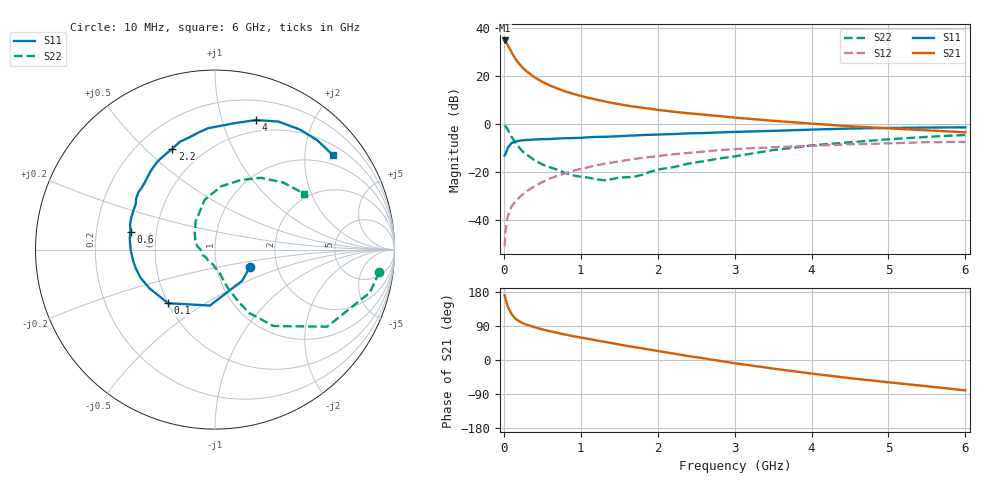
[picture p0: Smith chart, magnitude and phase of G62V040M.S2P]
! SIEMENS Small Signal Semiconductors
! BFG193
! Si NPN RF Bipolar Junction Transistor in SOT223
! VCE = 2 V  IC = 40 mA
! Common Emitter S-Parameters:  August  1996
# GHz  S  MA  R  50
!  f  S11  S21  S12  S22
! GHz  MAG  ANG  MAG  ANG  MAG  ANG  MAG  ANG
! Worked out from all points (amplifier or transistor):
!   36 points, 10 MHz to 6 GHz, reference 50 ohm
!   highest |S21| = 34.8 dB at 10 MHz (marker M1)
!   |S21| within 3 dB of that: start of sweep to 68.51 MHz
!   unconditionally stable (mu >= 1): 438.3 MHz to 2.559 GHz
!   at 250 MHz: K = 0.90, MSG = 26.3 dB, |S12| = -29.3 dB
!   at 1.4 GHz: K = 1.05, MAG = 11.1 dB, |S12| = -16.2 dB
!   at 6 GHz: K = 0.92, MSG = 2.0 dB, |S12| = -7.6 dB
!   S11 on the Smith chart (normalised r, x): 10 MHz: 1.45, -0.29; 100 MHz: 0.50, -0.36; 600 MHz: 0.35, +0.09; 2.2 GHz: 0.34, +0.61; 4 GHz: 0.38, +1.29; 6 GHz: 0.74, +2.67
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0.01  0.2173 -26.3  54.72 170.8  0.0028 83.9  0.9236 -7.8
0.02  0.2305 -48.8  52.69 162.9  0.0054 81.6  0.8957 -15.5
0.05  0.313 -95.2  44.17 141.5  0.0116 69.9  0.7583 -34.5
0.1  0.397 -131.2  30.99 121.5  0.0189 62.7  0.5359 -52.6
0.15  0.424 -149.4  22.63 109.1  0.0239 62.7  0.3994 -61.8
0.2  0.443 -159.1  17.81 102.3  0.0292 64.9  0.3183 -65.6
0.25  0.4533 -166.5  14.49 96.8  0.0341 65.2  0.2593 -69.1
0.3  0.4595 -171.7  12.26 92.8  0.0395 66.5  0.2247 -71.6
0.4  0.4694 -179.4  9.322 86.6  0.05 66.7  0.1733 -74.9
0.5  0.4785 173.1  7.495 80.7  0.0606 66.1  0.1419 -77.4
0.6  0.4809 168.2  6.291 75.9  0.0722 65.3  0.1238 -80.9
0.8  0.5 158.6  4.733 67.1  0.093 62.0  0.0946 -92.2
1.1  0.5232 147.1  3.475 55.6  0.1246 56.9  0.0754 -115.7
1.3  0.5344 140.1  2.95 48.2  0.1458 52.6  0.0664 -137.6
1.6  0.5637 129.8  2.401 37.2  0.1749 45.7  0.0767 -166.7
2.2  0.6103 112.9  1.788 17.2  0.2307 31.7  0.1244 152.4
2.8  0.6595 97.8  1.445 -2.1  0.2819 17.5  0.189 125.1
3.5  0.7112 81.6  1.155 -22.6  0.3244 0.0  0.2827 101.9
4  0.7567 72.5  1.009 -35.8  0.3461 -9.8  0.3536 84.6
4.5  0.7959 63.7  0.888 -48.0  0.374 -19.9  0.4125 69.9
5.5  0.8343 46.8  0.73 -69.3  0.4138 -42.9  0.5332 44.5
6  0.8423 38.6  0.664 -80.2  0.4174 -56.0  0.5855 32.2
